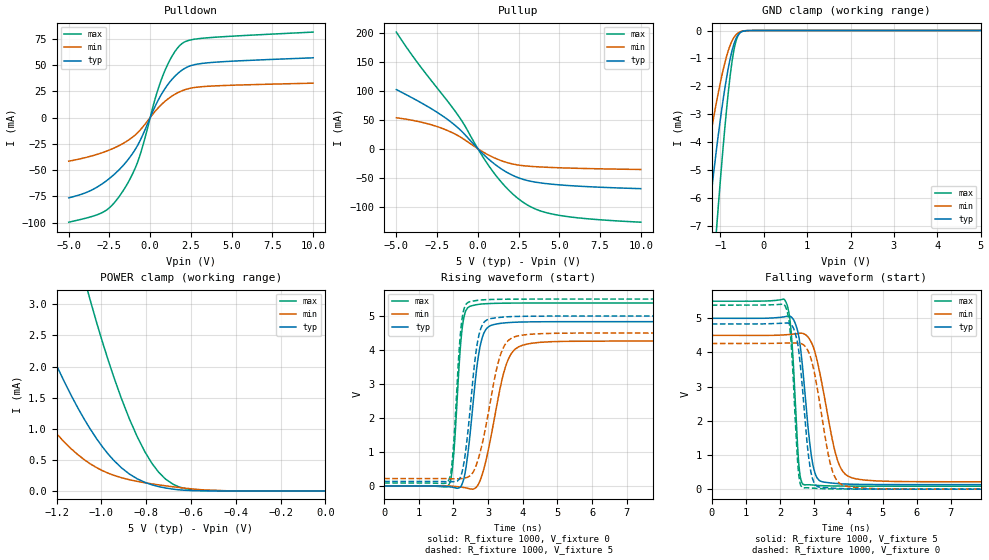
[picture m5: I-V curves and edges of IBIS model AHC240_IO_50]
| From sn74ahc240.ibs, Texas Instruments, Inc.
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[Model]   AHC240_IO_50
Model_type  3-state
Enable   Active-Low
Vref =   0
Rref =   1000
Cref =   50p
Vmeas =   2.5
| variable   typ   min   max
C_comp   2.08pF   1.91pF   2.16pF
| C_pullup   2.90pF   2.16pF   3.63pF
| C_pulldown   2.51pF   2.16pF   3.06pF
| C_tri-state   2.08pF   1.91pF   2.16pF
[Temperature Range]   40   100   -40
| Ambient temperature   25   85   -40
[Voltage range]   5   4.5   5.5
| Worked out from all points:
|   slope of the pulldown table from 0 to 0.75 V, typ, clamps not added: 31.8 ohm
|   slope of the pullup table from 0 to 0.75 V, typ, clamps not added: 37.1 ohm
|   GND clamp passes 1 mA (typ) near -0.77 V on its own axis
|   POWER clamp passes 1 mA (typ) near -1.05 V on its own axis
|   rising waveform, R_fixture 1000, V_fixture 0: 20-80 % time 309ps typ, 512ps min, 200ps max; typ from 0 V to 4.83 V
|   falling waveform, R_fixture 1000, V_fixture 5: 20-80 % time 289ps typ, 505ps min, 179ps max; typ from 5 V to 0.132 V
|   rising waveform, R_fixture 1000, V_fixture 5: 20-80 % time 301ps typ, 504ps min, 196ps max; typ from 0.132 V to 5 V
|   falling waveform, R_fixture 1000, V_fixture 0: 20-80 % time 267ps typ, 442ps min, 176ps max; typ from 4.83 V to 0 V
[GND Clamp]
| AHC240_IO_50
|   Voltage   I(typ)   I(min)   I(max)
-5V       -86.37mA   -56.48mA   -109.4mA
-1.55V    -11.02mA   -6.97mA    -17.41mA
-1.295V   -7.045mA   -4.381mA   -11.51mA
-1.09V    -4.251mA   -2.557mA   -7.121mA
-1.065V   -3.94mA    -2.355mA   -6.615mA
-890mV    -1.994mA   -1.11mA    -3.348mA
-775mV    -1.008mA   -526.3uA   -1.617mA
-675mV    -421.1uA   -217.2uA   -596.1uA
-630mV    -250.8uA   -134.3uA   -324.3uA
-560mV    -92.93uA   -56.51uA   -100.9uA
-360mV    -2.308uA   -1.765uA   -1.106uA
5V        33.38nA    7.111uA    302nA
[POWER Clamp]
| AHC240_IO_50
|   Voltage   I(typ)   I(min)   I(max)
-5V       75.68mA    48.36mA    122.9mA
-1.595V   5.897mA    3.159mA    12.53mA
-1.345V   3.264mA    1.609mA    7.646mA
-1.315V   2.988mA    1.452mA    7.117mA
-1.195V   1.981mA    900.5uA    5.136mA
-1.075V   1.146mA    499uA      3.399mA
-1.05V    997.6uA    437uA      3.071mA
-945mV    493.1uA    251.9uA    1.836mA
-840mV    195.2uA    153.7uA    872.7uA
-715mV    48.24uA    82.85uA    195uA
-590mV    4.19uA     30.5uA     16.84uA
-84.45fV  33.38nA    1.976nA    458.3nA
[Pulldown]
| AHC240_IO_50
|   Voltage   I(typ)   I(min)   I(max)
-5V       -76.31mA   -41.49mA   -99.44mA
-3.795V   -70.39mA   -37.38mA   -94.97mA
-2.815V   -61.55mA   -32.72mA   -89.22mA
-2.255V   -54.65mA   -29.24mA   -81.86mA
-1.62V    -44.85mA   -24.23mA   -68.56mA
-695mV    -24.18mA   -13.22mA   -38.97mA
310mV     10.9mA     6.027mA    18.24mA
800mV     24.86mA    13.89mA    40.7mA
1.37V     36.81mA    20.71mA    59.05mA
1.935V    44.82mA    25.28mA    70.04mA
3.495V    51.91mA    29.63mA    75.68mA
10V       56.7mA     32.62mA    81.13mA
[Pullup]
| AHC240_IO_50
|   Voltage   I(typ)   I(min)   I(max)
-5V       102mA      53.4mA     201.3mA
-3.725V   83.08mA    47.34mA    149.4mA
-1.745V   48.07mA    29.93mA    77.91mA
-935mV    28.44mA    17.7mA     45.93mA
120mV     -3.537mA   -2.209mA   -5.603mA
885mV     -23.37mA   -14.19mA   -37.91mA
1.7V      -39.45mA   -23.13mA   -65.83mA
2.515V    -50.46mA   -28.35mA   -87.03mA
3.525V    -57.7mA    -31.04mA   -104.1mA
4.76V     -61.86mA   -32.71mA   -113.9mA
6.77V     -65.58mA   -34.32mA   -121.1mA
10V       -69.01mA   -35.9mA    -126.9mA
[Ramp]
| AHC240_IO_50
| variable   typ   min   max
dV/dt_r   2.94/3.19E-10   2.62/5.26E-10   3.25/2.05E-10
dV/dt_f   2.96/2.96E-10   2.61/5.19E-10   3.29/1.86E-10
R_load = 1000
[Rising Waveform]
| AHC240_IO_50
R_fixture =   1000
C_fixture =   0
L_fixture =   0
V_fixture =   0
V_fixture_min = 0
V_fixture_max = 0
|   Time   V(typ)   V(min)   V(max)
0s        2.035nV    3.367nV    1.286nV
1.885ns   -28.01mV   -4.658mV   66.63mV
2.01ns    -47.79mV   -13.08mV   953.7mV
2.195ns   -38.57mV   -33.12mV   4.015V
2.29ns    174.1mV    -47.3mV    4.901V
2.795ns   4.225V     226.1mV    5.352V
2.99ns    4.666V     978.9mV    5.366V
3.58ns    4.807V     3.719V     5.38V
4.485ns   4.832V     4.225V     5.384V
50ns      4.835V     4.264V     5.385V
[Falling Waveform]
| AHC240_IO_50
R_fixture =   1000
C_fixture =   0
L_fixture =   0
V_fixture =   5
V_fixture_min = 4.5
V_fixture_max = 5.5
|   Time   V(typ)   V(min)   V(max)
0s        5V         4.5V       5.5V
2.165ns   5.051V     4.518V     5.487V
2.33ns    5.036V     4.532V     4.526V
2.56ns    4.395V     4.561V     605.8mV
2.73ns    2.792V     4.529V     122.9mV
2.91ns    1.014V     4.304V     125mV
3.085ns   325.6mV    3.759V     110.6mV
3.725ns   160.9mV    728.5mV    91.59mV
4.53ns    137.8mV    260.9mV    87.25mV
50ns      132.5mV    215.7mV    86mV
[Rising Waveform]
| AHC240_IO_50
R_fixture =   1000
C_fixture =   0
L_fixture =   0
V_fixture =   5
V_fixture_min = 4.5
V_fixture_max = 5.5
|   Time   V(typ)   V(min)   V(max)
0s        132.5mV    215.7mV    86mV
1.855ns   121.5mV    213mV      152.5mV
1.98ns    123.5mV    209.7mV    905.3mV
2.165ns   197.2mV    209.7mV    3.999V
2.265ns   480.9mV    218.2mV    5.019V
2.735ns   4.432V     855.9mV    5.467V
2.905ns   4.84V      1.598V     5.48V
3.41ns    4.967V     4V         5.494V
4.235ns   4.995V     4.465V     5.499V
50ns      5V         4.5V       5.5V
[Falling Waveform]
| AHC240_IO_50
R_fixture =   1000
C_fixture =   0
L_fixture =   0
V_fixture =   0
V_fixture_min = 0
V_fixture_max = 0
|   Time   V(typ)   V(min)   V(max)
0s        4.835V     4.264V     5.385V
2.15ns    4.861V     4.274V     5.356V
2.3ns     4.841V     4.276V     4.57V
2.47ns    4.463V     4.274V     1.555V
2.555ns   3.969V     4.271V     349.4mV
2.67ns    2.769V     4.233V     39.11mV
3.01ns    158.1mV    3.378V     25.78mV
3.555ns   29.25mV    468.8mV    7.303mV
4.23ns    7.029mV    44.9mV     2.075mV
50ns      505.7pV    4.154nV    612.6pV
